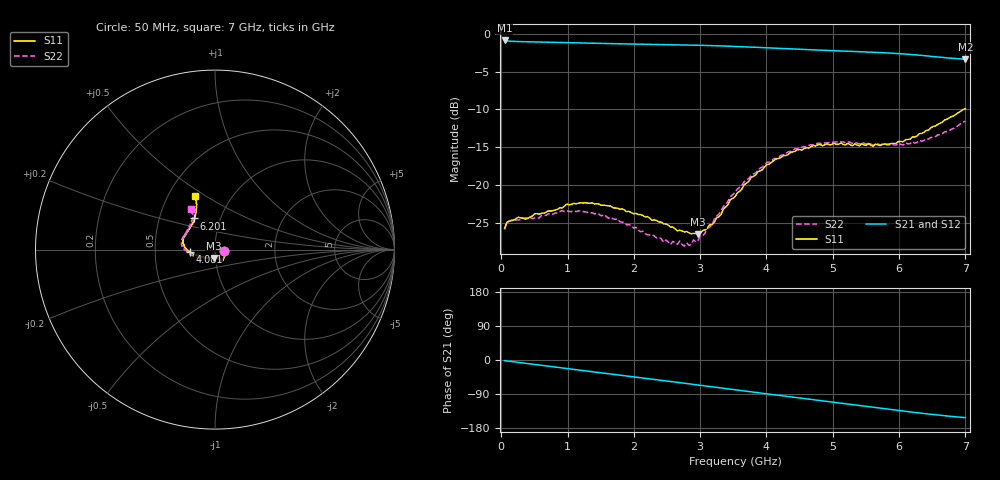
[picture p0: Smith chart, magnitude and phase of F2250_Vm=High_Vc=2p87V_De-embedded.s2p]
! Integrated Device Technology
! Corporate Headquarters
! 6024 Silver Creek Valley Road
! San Jose, CA 95138  USA
! Phone:  1-408-284-8200
! Toll Free:  1-800-223-1366
! Webpage:  http://www.idt.com/
! Timing and RF Division
! 515 Groton Road, Suite 102
! Westford, MA 01886-6024
! Device:  F2250
! Description: Voltage Variable RF Attenuator
! Frequency:  50.0 -  6000.00 MHz
! Package:  3x3 mm Thin QFN Plastic Package: 16 pin
! Ports:  2 RF, 3 DC
!  Pin  1  = GND
!  Pin  2  = NC
!  Pin  3  = RF1  = Port 1
!  Pin  4  = NC
!  Pin  5  = GND
!  Pin  6  = GND
!  Pin  7  = GND
!  Pin  8  = GND
!  Pin  9  = NC
!  Pin 10  = RF2  = Port 2
!  Pin 11  = NC
!  Pin 12  = GND
!  Pin 13  = GND
!  Pin 14  = VCNTRL
!  Pin 15  = VDD
!  Pin 16  = VMODE
! Vcntrl:  2.870 Volts
! Vmode:  +3.300 Volts
! Vdd:  +3.30  Volts
! Current:  1.310 mA
! Data:  The device was measured on a the F2250 evaluation board which has
!  individual transmission lines to the RF pins.  Data was collected
!  using a calibrated network analyzer.  The evaluation board was
!  de-embedded using a TRL calibration technique.
!  The reference plane is the edge of the package pin.
! Misc:  SN 10
!  Action Tracker AT0258
! Date Measured:  2014-11-26
! Date:  2015-10-15  MJV
! Note:
!  Integrated Device Technology supplies this data as a sample of measured
!  data at the package pin for this product.  Your particular data for this
!  product may vary.
!  Data was taken at 25 degrees C.
!  Integrated Device Technology reserves the right to change this data at anytime.
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# GHz S dB R 50
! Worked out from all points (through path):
!   201 points, 50 MHz to 7 GHz, reference 50 ohm
!   highest |S21| = -0.89 dB at 50 MHz (marker M1); lowest = -3.4 dB at 7 GHz (marker M2)
!   group delay of S21, straight-line fit = 61.1 ps
!   lowest |S11| = -26.5 dB at 2.969 GHz (marker M3), VSWR 1.10, Z = 49.1 - j4.63 ohm
!   |S11| at or under -10 dB: start of sweep to 6.967 GHz
!   |S22| runs from -28.0 to -11.5 dB; largest |S21 - S12| = 0.002
!   S11 on the Smith chart (normalised r, x): 50 MHz: 1.11, -0.02; 4.081 GHz: 0.75, -0.02; 6.201 GHz: 0.75, +0.27; 7 GHz: 0.68, +0.45
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0.05  -25.69 -10.8  -0.89 -1.8  -0.89 -1.8  -25.84 -11.0
0.1195  -24.76 -10.1  -0.99 -3.2  -0.98 -3.2  -24.70 -8.8
0.57125  -23.84 -31.3  -1.10 -13.3  -1.10 -13.3  -24.33 -31.4
0.91875  -23.00 -50.1  -1.17 -21.0  -1.17 -21.1  -23.35 -51.0
1.2315  -22.36 -57.9  -1.24 -27.9  -1.24 -27.9  -23.47 -61.5
1.75275  -23.03 -64.8  -1.33 -39.1  -1.33 -39.1  -24.42 -67.8
2.37825  -24.86 -64.5  -1.42 -52.8  -1.42 -52.8  -26.87 -66.7
2.552  -25.51 -69.5  -1.44 -56.7  -1.44 -56.7  -27.84 -73.1
2.691  -25.92 -77.5  -1.47 -59.8  -1.47 -59.8  -27.37 -80.8
2.7605  -26.17 -79.7  -1.48 -61.3  -1.48 -61.3  -28.04 -85.3
2.969  -26.48 -97.8  -1.52 -66.0  -1.52 -66.0  -27.27 -104.8
3.1775  -25.20 -120.9  -1.57 -70.7  -1.57 -70.7  -25.25 -126.7
3.525  -21.54 -152.8  -1.68 -78.5  -1.68 -78.6  -20.97 -148.7
3.76825  -18.96 -164.8  -1.77 -84.0  -1.77 -84.1  -18.69 -159.6
4.081  -16.95 -175.7  -1.90 -91.0  -1.90 -91.0  -16.72 -171.4
4.4285  -15.54 176.0  -2.03 -98.6  -2.04 -98.7  -15.20 178.7
4.7065  -14.76 169.1  -2.13 -104.8  -2.13 -104.8  -14.68 173.0
5.054  -14.60 160.9  -2.26 -112.5  -2.25 -112.5  -14.27 166.0
5.85325  -14.57 135.1  -2.56 -130.0  -2.56 -130.1  -14.67 147.3
6.20075  -13.62 123.5  -2.77 -137.7  -2.77 -137.8  -14.25 138.2
6.54825  -12.18 115.6  -3.04 -144.7  -3.04 -144.9  -13.58 126.9
7  -9.91 110.7  -3.37 -152.1  -3.37 -152.2  -11.54 120.7
